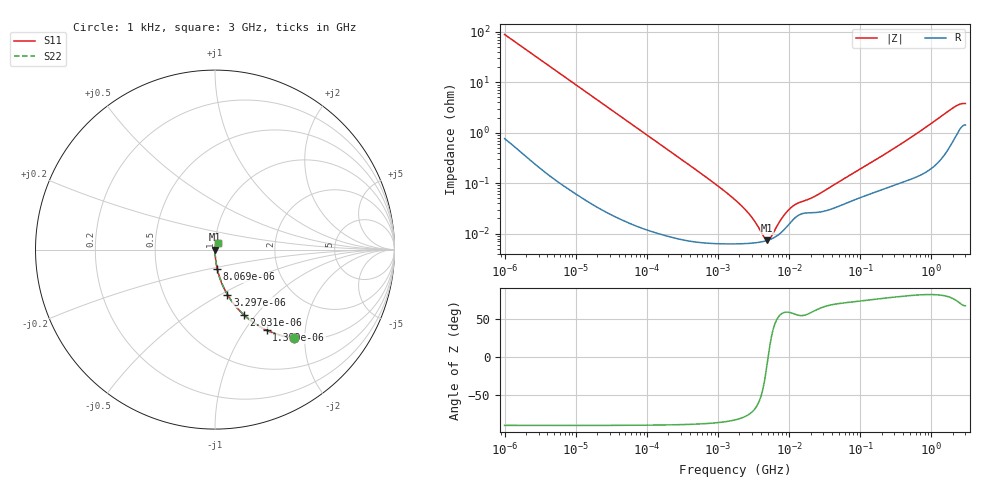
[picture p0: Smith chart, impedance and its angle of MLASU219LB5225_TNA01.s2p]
! MLASU219LB5225_TNA01  S-PARAMETER MODEL  ( Standard Model )
! Model Generated by TAIYO YUDEN Corporation (http://www.ty-top.com)
! Version 1.0
! TAIYO YUDEN Control No. 220601
! Copyright(c) 2012 TAIYO YUDEN CO.,LTD. All Rights Reserved.
! Product Description (link to TY-COMPAS)
! https://ds.yuden.co.jp/TYCOMPAS/or/detail?pn=MLASU219LB5225KTNA01&u=M
! Products Name : Multilayer Ceramic Capacitors
! Characteristics :
!  Capacitance : 2.2 [uF] , Rated Voltage : 50 [V] , TCC : X5R
!  Case Size : 2.0 x 1.25 / 0.079 x 0.049 [mm/inch] , Thickness : 0.85 / 0.033 [mm/inch]
!  (Conditions: Temperature = 25 [degC] , DC Bias Voltage = 0 [V])
! External Node Assignments :
!  1  o---| |---o  2
! GND o---------o GND
! Frequency Range : 1kHz  -  3GHz  [ 401 STEP ]
# MHZ S RI R 50
! Freq[MHz].  S11 Real  S11 Imag  S21 Real  S21 Imag  S12 Real  S12 Imag  S22 Real  S22 Imag
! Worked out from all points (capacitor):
!   401 points, 1 kHz to 3 GHz, reference 50 ohm
!   read as one part in series: C = 1.79 uF near 1.077 kHz
!   lowest |Z| = 7.39 mohm at 4.92 MHz (marker M1)
!   series resonance near 5.054 MHz, so ESL is about 550 pH
!   S11 on the Smith chart (normalised r, x): 1 kHz: 1.02, -1.77; 1.399 kHz: 1.01, -1.27; 2.031 kHz: 1.01, -0.88; 3.297 kHz: 1.00, -0.54; 8.069 kHz: 1.00, -0.22; 3 GHz: 1.03, +0.07
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0.001  0.4397 -0.4921  0.5603 0.4921  0.5603 0.4921  0.4397 -0.4921
0.001399  0.2883 -0.4489  0.7117 0.4489  0.7117 0.4489  0.2883 -0.4489
0.002031  0.1626 -0.3652  0.8374 0.3652  0.8374 0.3652  0.1626 -0.3652
0.003297  0.0695 -0.2508  0.9305 0.2508  0.9305 0.2508  0.0695 -0.2508
0.008069  0.0128 -0.1092  0.9872 0.1092  0.9872 0.1092  0.0128 -0.1092
0.01216  0.00589 -0.0731  0.9941 0.0731  0.9941 0.0731  0.00589 -0.0731
0.033275  0.000954 -0.027  0.999 0.027  0.999 0.027  0.000954 -0.027
0.147855  0.000136 -0.00611  0.9999 0.00611  0.9999 0.00611  0.000136 -0.00611
0.791611  6.52e-05 -0.00112  0.9999 0.00112  0.9999 0.00112  6.52e-05 -0.00112
1.732051  6.28e-05 -0.000465  0.9999 0.000465  0.9999 0.000465  6.28e-05 -0.000465
2.812335  6.43e-05 -0.000225  0.9999 0.000225  0.9999 0.000225  6.43e-05 -0.000225
4.083148  6.86e-05 -7.87e-05  0.9999 7.87e-05  0.9999 7.87e-05  6.86e-05 -7.87e-05
4.399271  7.02e-05 -5.1e-05  0.9999 5.1e-05  0.9999 5.1e-05  7.02e-05 -5.1e-05
4.919932  7.32e-05 -9.83e-06  0.9999 9.83e-06  0.9999 9.83e-06  7.32e-05 -9.83e-06
5.928204  8.13e-05 5.95e-05  0.9999 -5.95e-05  0.9999 -5.95e-05  8.13e-05 5.95e-05
8.291982  0.000116 0.00019  0.9999 -0.00019  0.9999 -0.00019  0.000116 0.00019
11.1738  0.000184 0.000294  0.9998 -0.000294  0.9998 -0.000294  0.000184 0.000294
21.06097  0.00026 0.000446  0.9997 -0.000446  0.9997 -0.000446  0.00026 0.000446
256.0921  0.000859 0.00419  0.9991 -0.00419  0.9991 -0.00419  0.000859 0.00419
2066.299  0.00818 0.0306  0.9918 -0.0306  0.9918 -0.0306  0.00818 0.0306
2489.759  0.0126 0.0339  0.9874 -0.0339  0.9874 -0.0339  0.0126 0.0339
3000  0.0152 0.0341  0.9848 -0.0341  0.9848 -0.0341  0.0152 0.0341
